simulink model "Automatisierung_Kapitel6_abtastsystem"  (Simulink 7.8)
settings: Solver=ode45  StartTime=0.0  StopTime=5  MaxStep=0.2  RelTol=1e-3
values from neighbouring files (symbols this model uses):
  Ac = [-2,1;-1,-2]    [Automatisierung_Kapitel6.m]
  bc = [0,1]'    [Automatisierung_Kapitel6.m]
  cc = [1,0]    [Automatisierung_Kapitel6.m]
  dc = 1    [Automatisierung_Kapitel6.m]
  TA1 = 0.2    [Automatisierung_Kapitel6.m]
libraries: cstblocks x1

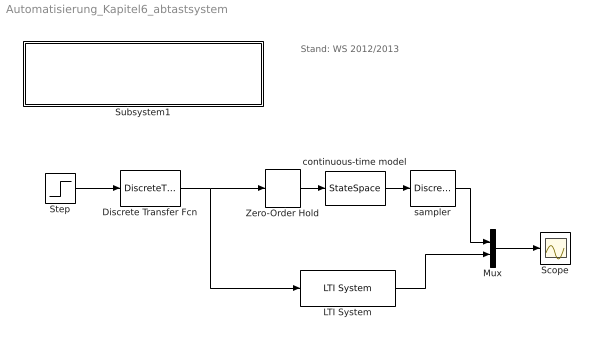
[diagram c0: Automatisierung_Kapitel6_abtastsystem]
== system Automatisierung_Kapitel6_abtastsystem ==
  note: Stand: WS 2012/2013
  Discrete Transfer Fcn : DiscreteTransferFcn  Denominator=[1 -0.5]  SampleTime=TA1
  LTI System : cstblocks/LTI System  sys=sysD  IC=[0,0]
  Mux : Mux  Inputs=2
  Scope : Scope
  Step : Step  Time=0  SampleTime=0
  Subsystem1 : Subsystem  Description=asas
  Zero-Order Hold : ZeroOrderHold  SampleTime=TA1
  continuous-time model : StateSpace  A=Ac  B=bc  C=cc  D=dc  X0=[0,0]
  sampler : DiscreteTransferFcn  Denominator=[1]  SampleTime=TA1
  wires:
  Zero-Order Hold/1 -> continuous-time model/1
  continuous-time model/1 -> sampler/1
  sampler/1 -> Mux/1
  LTI System/1 -> Mux/2
  Mux/1 -> Scope/1
  Step/1 -> Discrete Transfer Fcn/1
  Discrete Transfer Fcn/1 -> Zero-Order Hold/1, LTI System/1

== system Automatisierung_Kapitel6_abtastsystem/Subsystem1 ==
